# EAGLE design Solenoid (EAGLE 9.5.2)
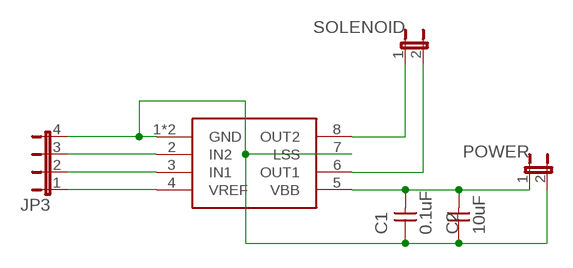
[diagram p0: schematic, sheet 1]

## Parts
C1  0.1uF  CAP_UNPOLARIZEDFAB  [C1206FAB]
C2  10uF  CAP_UNPOLARIZEDFAB  [C1206FAB]
JP3  JP4E  [JP4]
POWER  JP1E  [JP1]
SOLENOID  JP1E  [JP1]
U$1  PMIC_H-BRIDGE_A4953_PAD  [SOIC8_PAD]

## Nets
N$1: C1.1 C2.1 JP3.4 POWER.2 U$1.1(GND) U$1.7(LSS) U$1.GND
N$2: JP3.3 U$1.2(IN2)
N$3: JP3.2 U$1.3(IN1)
N$4: JP3.1 U$1.4(VREF)
N$5: C1.2 C2.2 POWER.1 U$1.5(VBB)
N$6: SOLENOID.1 U$1.8(OUT2)
N$7: SOLENOID.2 U$1.6(OUT1)

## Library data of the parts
C1 C2 = fab:CAP_UNPOLARIZED
JP3 = jumper:JP4E: JUMPER
POWER SOLENOID = jumper:JP1E: JUMPER
U$1 = fab:PMIC_H-BRIDGE_A4953_PAD

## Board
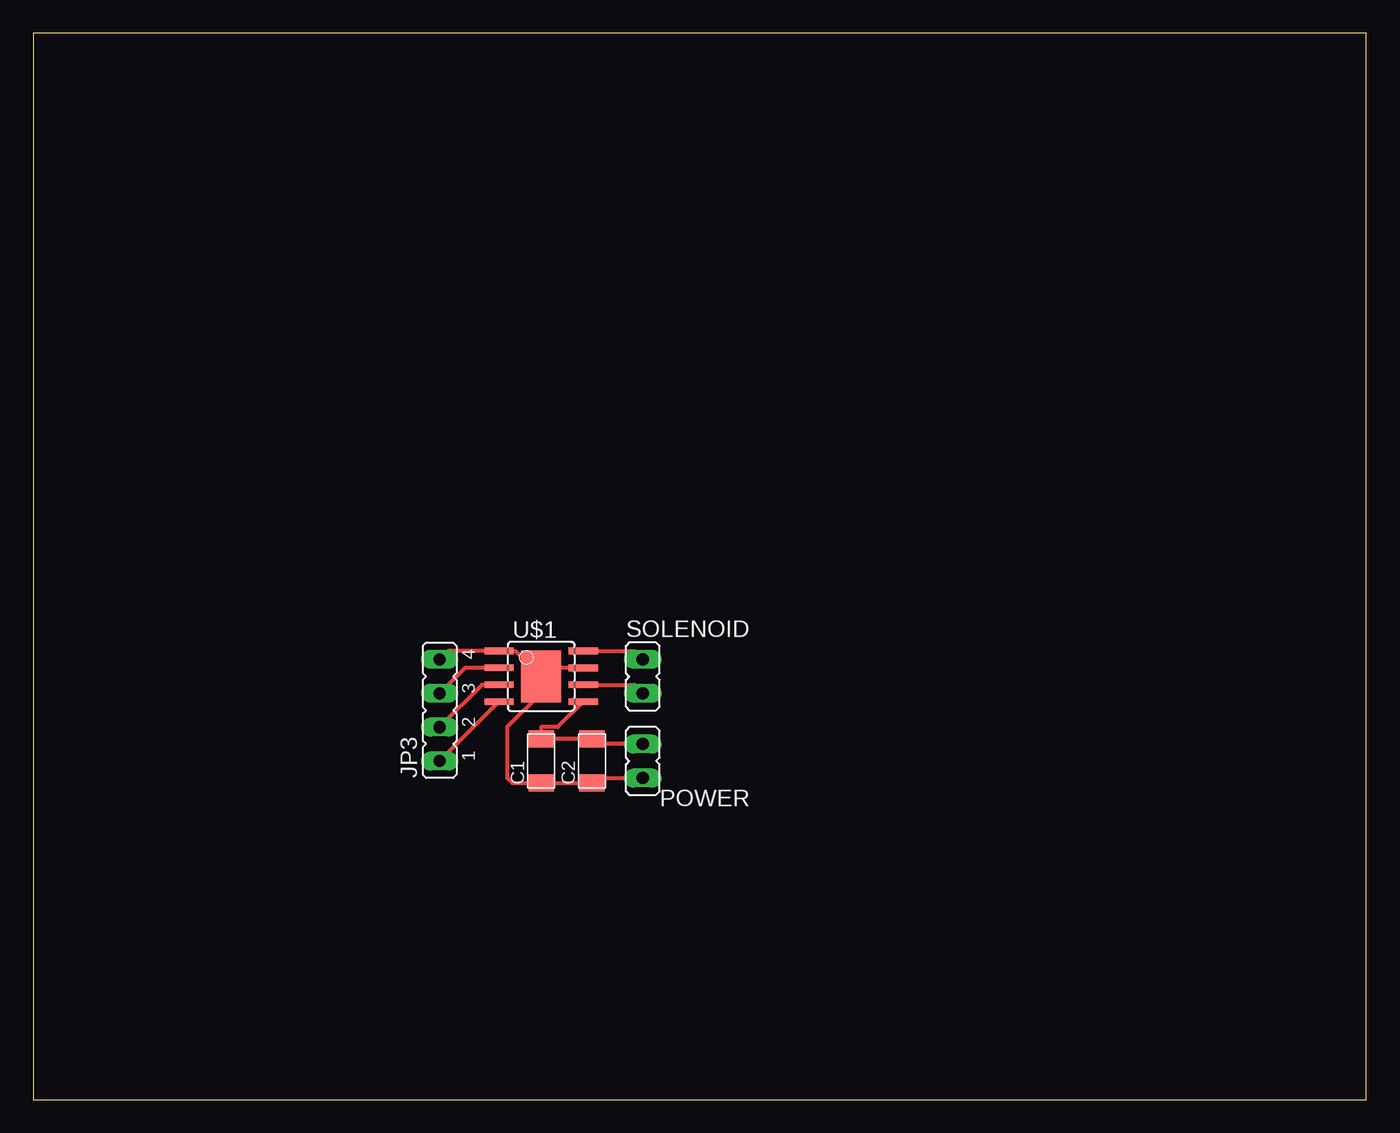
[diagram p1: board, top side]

Size 100 x 80 mm. Coordinates in mm from the lower left corner, seen from the top.
Outline: 0,0 100,0 100,80 0,80 0,0
Copper layers (1*16): Top 0.035mm / dielectric 1.5mm / Bottom 0.035mm
Design rules "default *": minimum track width 12mil, minimum drill 32mil, track to track 16mil, track to pad 16mil, pad to pad 16mil, via to via 16mil, smd to smd 16mil, copper to edge 16mil, drill to drill 16mil, minimum pad ring 10mil, minimum via ring 8mil, stop-mask expansion 4mil, vias tented up to drill 0mil, thermal gap 10mil

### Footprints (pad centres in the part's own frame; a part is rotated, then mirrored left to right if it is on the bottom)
C1206FAB = smd 1.27 x 1.905: 1 -1.651,0; 2 1.651,0
JP4 = drill 0.914 long: 1 -3.81,0; 2 -1.27,0; 3 1.27,0; 4 3.81,0
JP1 = drill 0.914 long: 1 0,-1.27; 2 0,1.27
SOIC8_PAD = smd 0.5 x 2.2: 1 -1.905,-3.154; 2 -0.645,-3.154; 3 0.625,-3.154; 4 1.895,-3.154; 5 1.905,3.154; 6 0.635,3.154; 7 -0.635,3.154; 8 -1.905,3.154 | smd 3.886 x 2.997: GND 0,0

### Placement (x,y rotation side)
C1  38.1,25.4 90 top
C2  41.91,25.4 90 top
JP3  30.48,29.21 90 top
POWER  45.72,25.4 180 top
SOLENOID  45.72,31.75 180 top
U$1  38.1,31.75 270 top

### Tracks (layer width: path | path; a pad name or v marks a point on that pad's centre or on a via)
N$1
  Top 0.305: U$1.GND 36.2,33.66 U$1.1 31.11,33.66 JP3.4 | 36.83,30.48 U$1.GND | U$1.7 38.73,32.38 U$1.GND | U$1.GND 38.1,30.48 35.56,27.94 35.56,24.13 35.94,23.75 C1.1 C2.1 42.29,24.13 POWER.2
N$2
  Top 0.305: U$1.2 32.4,32.4 JP3.3
N$3
  Top 0.305: U$1.3 33.66,31.12 JP3.2
N$4
  Top 0.305: U$1.4 JP3.1
N$5
  Top 0.305: POWER.1 42.29,26.67 C2.2 C1.2 38.1,27.94 39.35,27.94 U$1.5
N$6
  Top 0.305: U$1.8 45.09,33.66 SOLENOID.1
N$7
  Top 0.305: U$1.6 45.09,31.11 SOLENOID.2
